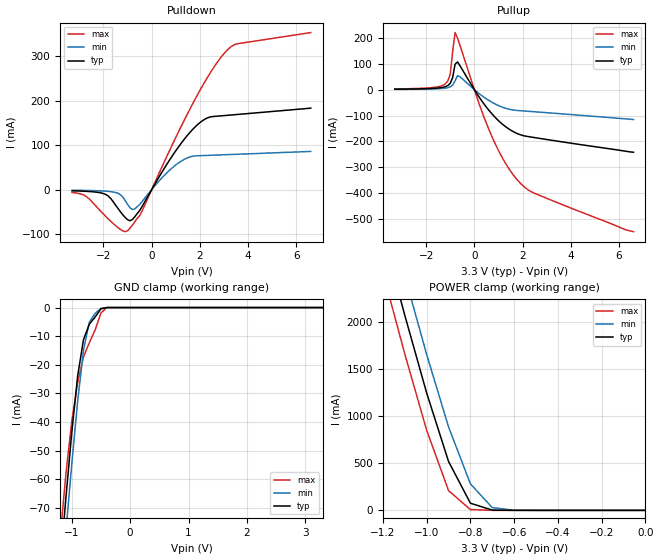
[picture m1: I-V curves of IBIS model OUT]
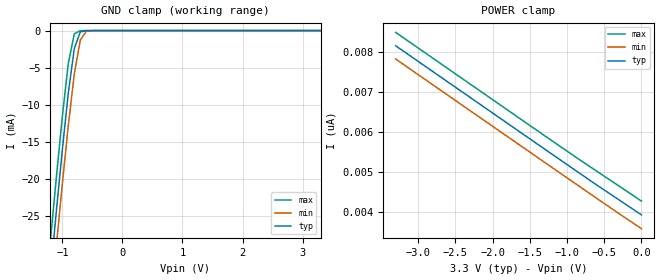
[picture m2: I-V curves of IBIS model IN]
|   TEXAS INSTRUMENTS INCORPORATED
|   Standard Linear and Logic
|   IBIS Model of SN74ALVC16334
|   16-BIT Universal Bus Driver with 3-state outputs
|   48-pin DGG, DGV, or DL Package
[IBIS Ver]   2.1
[Comment char]  |_char
[File Name]   alvc16334.ibs
[File Rev]   2.0
[Date]   9/29/98
[Source]   File originated at Texas Instruments, Inc.
[Notes]   The following is an IBIS list for the ALVC16334.
|   - This file may be incomplete or may not be fully compliant
|   with the IBIS specification. It will be replaced with a
|   version that is IBIS Revision 3.2 compliant and is complete
|   and accurate.  Please email all questions and comments to
|   sllibis@ti.com.
|   - All test data contained in this file are derived from
|   hspice(tm) simulations.
|   - File created by David Yaeger, SLL Applications
[Disclaimer]
* Property of Texas Instruments Incorporated.  Unauthorized *
* reproduction and/or distribution is strictly prohibited. *
* This product is protected under copyright law. *
* Created 1997, (C) Copyright 1997, Texas Instruments Inc., *
* All Rights Reserved *
* UNLESS THERE IS A SIGNED, WRITTEN AGREEMENT TO THE *
* CONTRARY, TEXAS INSTRUMENTS ("TI") IS PROVIDING THE IBIS *
* MODELS "AS IS" AND WITHOUT ANY WARRANTY, EXPRESSED OR *
* IMPLIED.  TI assumes no liability for: *
* 1) the accuracy of the IBIS models provided to your *
* company; *
* 2) the proper functioning of these IBIS models in your *
* design or for any resulting applications; or *
* 3) infringement of patents, copyrights or intellectual *
* property rights resulting from your use of these *
* IBIS models. *
* TI provides IBIS Models as a service to our customers. *
* You and your company shall not distribute, sell or give *
* these models to anyone else without prior written *
* permission from TI. *
* TI reserves the right to make changes to our products or *
* to discontinue any semiconductor product or service *
* without notice, and advises our customers to obtain the *
* latest version of relevant information to verify, before *
* placing orders, that the information being relied on is *
* current. *
* Please be aware that your receipt and use of the IBIS *
* information provided shall serve as acceptance of these *
* terms and conditions.  If you do not accept these terms, *
* you should return or destroy the IBIS models and any *
* other accompanying information immediately. *
[Component]   ALVC16334_DGG
[Manufacturer]  Texas Instruments, Inc.
[Package]
|   typ   min   max
R_pkg   0.056   0.039   0.068
L_pkg   3.39nH   3.078nH   3.995nH
C_pkg   0.52pF   0.414pF   0.668pF
[Pin]   signal_name   model_name   R_pin   L_pin   C_pin
1   OE_BAR   NC   0.039   3.987nH   0.654pF
2   Y1   OUT   0.047   3.725nH   0.659pF
3   Y2   OUT   0.059   3.692nH   0.604pF
4   GND   GND   0.068   3.675nH   0.606pF
5   Y3   OUT   0.055   3.473nH   0.547pF
6   Y4   OUT   0.056   3.402nH   0.497pF
7   VCC   POWER   0.057   3.3nH   0.492pF
8   Y5   OUT   0.056   3.189nH   0.455pF
9   Y6   OUT   0.058   3.154nH   0.449pF
10   GND   GND   0.058   3.094nH   0.436pF
11   Y7   OUT   0.058   3.078nH   0.424pF
12   Y8   OUT   0.06   3.081nH   0.414pF
13   Y9   OUT   0.061   3.097nH   0.416pF
14   Y10   OUT   0.06   3.126nH   0.427pF
15   GND   GND   0.061   3.158nH   0.44pF
16   Y11   OUT   0.058   3.173nH   0.45pF
17   Y12   OUT   0.056   3.189nH   0.455pF
18   VCC   POWER   0.056   3.265nH   0.49pF
19   Y13   OUT   0.054   3.322nH   0.492pF
20   Y14   OUT   0.052   3.388nH   0.544pF
21   GND   GND   0.064   3.591nH   0.605pF
22   Y15   OUT   0.059   3.677nH   0.612pF
23   Y16   OUT   0.046   3.678nH   0.668pF
24   NC   NC   0.041   3.979nH   0.659pF
25   LE_BAR   NC   0.04   3.995nH   0.658pF
26   A16   IN   0.046   3.69nH   0.662pF
27   A15   IN   0.057   3.649nH   0.602pF
28   GND   GND   0.066   3.615nH   0.602pF
29   A14   IN   0.055   3.447nH   0.547pF
30   A13   IN   0.054   3.326nH   0.492pF
31   VCC   POWER   0.055   3.239nH   0.488pF
32   A12   IN   0.056   3.183nH   0.454pF
33   A11   IN   0.057   3.144nH   0.447pF
34   GND   GND   0.058   3.099nH   0.436pF
35   A10   IN   0.059   3.086nH   0.425pF
36   A9   IN   0.06   3.081nH   0.414pF
37   A8   IN   0.061   3.097nH   0.415pF
38   A7   IN   0.06   3.119nH   0.427pF
39   GND   GND   0.06   3.144nH   0.439pF
40   A6   IN   0.056   3.13nH   0.446pF
41   A5   IN   0.057   3.208nH   0.456pF
42   VCC   POWER   0.056   3.247nH   0.487pF
43   A4   IN   0.054   3.328nH   0.491pF
44   A3   IN   0.053   3.413nH   0.546pF
45   GND   GND   0.066   3.609nH   0.606pF
46   A2   IN   0.058   3.689nH   0.607pF
47   A1   IN   0.047   3.727nH   0.662pF
48   CLK   NC   0.04   3.978nH   0.655pF
[Component]   ALVC16334_DGV
[Manufacturer]  Texas Instruments, Inc.
[Package]
|   typ   min   max
R_pkg   0.063   0.043   0.09
L_pkg   3.077nH   2.377nH   4.305nH
C_pkg   0.387pF   0.281pF   0.565pF
[Pin]   signal_name   model_name   R_pin   L_pin   C_pin
1   OE_BAR   NC   0.082   4.277nH   0.562pF
2   Y1   OUT   0.09   4.02nH   0.554pF
3   Y2   OUT   0.087   3.719nH   0.478pF
4   GND   GND   0.087   3.456nH   0.417pF
5   Y3   OUT   0.076   3.207nH   0.411pF
6   Y4   OUT   0.044   2.929nH   0.39pF
7   VCC   POWER   0.046   2.803nH   0.335pF
8   Y5   OUT   0.047   2.683nH   0.321pF
9   Y6   OUT   0.048   2.579nH   0.311pF
10   GND   GND   0.049   2.505nH   0.302pF
11   Y7   OUT   0.048   2.4nH   0.289pF
12   Y8   OUT   0.051   2.4nH   0.283pF
13   Y9   OUT   0.051   2.4nH   0.283pF
14   Y10   OUT   0.05   2.433nH   0.291pF
15   GND   GND   0.048   2.46nH   0.298pF
16   Y11   OUT   0.048   2.585nH   0.312pF
17   Y12   OUT   0.046   2.652nH   0.319pF
18   VCC   POWER   0.045   2.787nH   0.336pF
19   Y13   OUT   0.046   2.962nH   0.394pF
20   Y14   OUT   0.074   3.208nH   0.409pF
21   GND   GND   0.087   3.488nH   0.417pF
22   Y15   OUT   0.087   3.741nH   0.478pF
23   Y16   OUT   0.089   3.99nH   0.546pF
24   NC   NC   0.084   4.305nH   0.557pF
25   LE_BAR   NC   0.082   4.286nH   0.565pF
26   A16   IN   0.086   3.933nH   0.554pF
27   A15   IN   0.086   3.699nH   0.475pF
28   GND   GND   0.089   3.522nH   0.42pF
29   A14   IN   0.079   3.234nH   0.413pF
30   A13   IN   0.043   2.88nH   0.385pF
31   VCC   POWER   0.045   2.779nH   0.332pF
32   A12   IN   0.045   2.636nH   0.317pF
33   A11   IN   0.047   2.553nH   0.309pF
34   GND   GND   0.048   2.468nH   0.298pF
35   A10   IN   0.05   2.424nH   0.29pF
36   A9   IN   0.05   2.377nH   0.281pF
37   A8   IN   0.05   2.387nH   0.281pF
38   A7   IN   0.05   2.431nH   0.29pF
39   GND   GND   0.048   2.475nH   0.299pF
40   A6   IN   0.048   2.557nH   0.309pF
41   A5   IN   0.047   2.671nH   0.319pF
42   VCC   POWER   0.046   2.804nH   0.334pF
43   A4   IN   0.044   2.935nH   0.39pF
44   A3   IN   0.074   3.203nH   0.412pF
45   GND   GND   0.085   3.444nH   0.416pF
46   A2   IN   0.085   3.723nH   0.477pF
47   A1   IN   0.09   4.012nH   0.547pF
48   CLK   NC   0.083   4.288nH   0.558pF
[Component]   ALVC16334_DL
[Manufacturer]  Texas Instruments, Inc.
[Package]
|   typ   min   max
R_pkg   0.048   0.038   0.053
L_pkg   6.046nH   5.084nH   7.968nH
C_pkg   0.813pF   0.569pF   1.157pF
[Pin]   signal_name   model_name   R_pin   L_pin   C_pin
1   OE_BAR   NC   0.046   7.968nH   1.017pF
2   Y1   OUT   0.044   7.299nH   1.157pF
3   Y2   OUT   0.043   6.765nH   1.058pF
4   GND   GND   0.041   6.269nH   0.933pF
5   Y3   OUT   0.038   5.856nH   0.829pF
6   Y4   OUT   0.046   5.802nH   0.79pF
7   VCC   POWER   0.05   5.656nH   0.738pF
8   Y5   OUT   0.053   5.5nH   0.643pF
9   Y6   OUT   0.052   5.304nH   0.606pF
10   GND   GND   0.053   5.189nH   0.583pF
11   Y7   OUT   0.051   5.084nH   0.569pF
12   Y8   OUT   0.053   5.862nH   0.833pF
13   Y9   OUT   0.053   5.862nH   0.833pF
14   Y10   OUT   0.051   5.084nH   0.569pF
15   GND   GND   0.053   5.189nH   0.583pF
16   Y11   OUT   0.052   5.304nH   0.606pF
17   Y12   OUT   0.053   5.5nH   0.643pF
18   VCC   POWER   0.05   5.656nH   0.738pF
19   Y13   OUT   0.046   5.802nH   0.79pF
20   Y14   OUT   0.038   5.856nH   0.829pF
21   GND   GND   0.041   6.269nH   0.933pF
22   Y15   OUT   0.043   6.765nH   1.058pF
23   Y16   OUT   0.044   7.299nH   1.157pF
24   NC   NC   0.046   7.968nH   1.017pF
25   LE_BAR   NC   0.046   7.968nH   1.017pF
26   A16   IN   0.044   7.299nH   1.157pF
27   A15   IN   0.043   6.765nH   1.058pF
28   GND   GND   0.041   6.269nH   0.933pF
29   A14   IN   0.038   5.856nH   0.829pF
30   A13   IN   0.046   5.802nH   0.79pF
31   VCC   POWER   0.05   5.656nH   0.738pF
32   A12   IN   0.053   5.5nH   0.643pF
33   A11   IN   0.052   5.304nH   0.606pF
34   GND   GND   0.053   5.189nH   0.583pF
35   A10   IN   0.051   5.084nH   0.569pF
36   A9   IN   0.053   5.862nH   0.833pF
37   A8   IN   0.053   5.862nH   0.833pF
38   A7   IN   0.051   5.084nH   0.569pF
39   GND   GND   0.053   5.189nH   0.583pF
40   A6   IN   0.052   5.304nH   0.606pF
41   A5   IN   0.053   5.5nH   0.643pF
42   VCC   POWER   0.05   5.656nH   0.738pF
43   A4   IN   0.046   5.802nH   0.79pF
44   A3   IN   0.038   5.856nH   0.829pF
45   GND   GND   0.041   6.269nH   0.933pF
46   A2   IN   0.043   6.765nH   1.058pF
47   A1   IN   0.044   7.299nH   1.157pF
48   CLK   NC   0.046   7.967nH   1.017pF
| Models and submodels in the file (2): OUT (3-state), IN (Input)
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|   Model ALVC16334_OUT
[Model]   OUT
Model_type   3-state
Polarity   Non-Inverting
Enable   Active-High
|Variable   typ   min   max
C_comp   7.0pF   NA   NA
[Voltage range]   3.3   3.0   3.6
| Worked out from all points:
|   slope of the pulldown table from 0 to 0.495 V, typ, clamps not added: 10.9 ohm
|   slope of the pullup table from 0 to 0.495 V, typ, clamps not added: 7.36 ohm
|   GND clamp passes 1 mA (typ) near -0.52 V on its own axis
|   POWER clamp passes 1 mA (typ) near -0.63 V on its own axis
[Pullup]   | Note: Vtable = Vcc - Voutput
|   Voltage   I(typ)   I(min)   I(max)
-3.3V     1.7mA      1mA        2.8mA
-1.2V     11.5mA     5.8mA      22.8mA
-1V       24.5mA     10.9mA     60.01mA
-900mV    46.68mA    17.53mA    148mA
-800mV    98.42mA    34.15mA    220.6mA
-700mV    107.1mA    53.45mA    199.3mA
-600mV    92.82mA    50.22mA    171.6mA
600mV     -79.52mA   -41.73mA   -153.4mA
1.2V      -136.3mA   -69.07mA   -270mA
1.8V      -170.6mA   -80.67mA   -350.9mA
2.5V      -185.4mA   -85.56mA   -400.8mA
6.6V      -242mA     -115.5mA   -548.8mA
[Pulldown]
|   Voltage   I(typ)   I(min)   I(max)
-3.3V     -2.523mA   -1.255mA   -6.217mA
-2.7V     -3.72mA    -1.71mA    -15.66mA
-1.9V     -10.77mA   -3.325mA   -60.13mA
-1.3V     -49.18mA   -11.05mA   -88.98mA
-1V       -67.21mA   -32.84mA   -92.31mA
-700mV    -60.66mA   -43.17mA   -72.11mA
800mV     71.29mA    46.5mA     94.49mA
1.7V      135.3mA    75.09mA    192.6mA
2.3V      160.9mA    76.98mA    250.7mA
3.1V      166.8mA    78.63mA    311.4mA
3.5V      168.6mA    79.46mA    327mA
6.6V      183.1mA    86mA       352.8mA
[POWER_Clamp]   | Note: Vtable = Vcc - Voutput
|   Voltage   I(typ)   I(min)   I(max)
-3.3V     22.55A     22.92A     22.19A
-1.2V     2.935A     3.354A     2.523A
-1.1V     2.069A     2.487A     1.659A
-1V       1.245A     1.653A     850.2mA
-900mV    518.9mA    885.7mA    209.9mA
-800mV    75.77mA    281.1mA    8.953mA
-700mV    2.801mA    29.05mA    160uA
-600mV    75.4uA     1.568mA    1.514uA
0V        990pA      903.2pA    1.08nA
[GND_Clamp]
|   Voltage   I(typ)   I(min)   I(max)
-3.3V     -640.3mA   -651.6mA   -629.4mA
-1.2V     -90.31mA   -102.4mA   -80.27mA
-1.1V     -66.22mA   -78.02mA   -57.91mA
-1V       -43.5mA    -54.54mA   -39.6mA
-900mV    -23.93mA   -32.78mA   -26.27mA
-800mV    -11.24mA   -14.93mA   -17.28mA
-700mV    -5.815mA   -5.06mA    -12.29mA
-600mV    -3.276mA   -2.035mA   -7.795mA
-500mV    -416.4uA   -247.1uA   -1.885mA
-400mV    -9.992nA   -367.3nA   -984.6pA
3.3V      990pA      123.6nA    930pA
[Ramp]
| variable   typ   min   max
dV/dt_r   1.7364E+00/1.9231E-10  1.3957E+00/2.9903E-10  2.0142E+00/1.7016E-10
dV/dt_f   1.6302E+00/2.0099E-10  1.3593E+00/4.4330E-10  1.8600E+00/1.6534E-10
|   Model ALVC16334_IN
[Model]   IN
Model_type   Input
Polarity   Non-Inverting
Vinl = 0.8V
Vinh = 2.0V
|Variable   typ   min   max
C_comp   6pF   NA   NA
[Voltage Range]   3.3   3.0   3.6
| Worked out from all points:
|   GND clamp passes 1 mA (typ) near -0.74 V on its own axis
[POWER_Clamp]   | Note: Vtable = Vcc - Voutput
|   Voltage   I(typ)   I(min)   I(max)
-3.3V     8.169nA    7.835nA    8.505nA
-1V       5.186nA    4.852nA    5.523nA
-600mV    4.672nA    4.336nA    5.018nA
0V        3.921nA    3.575nA    4.268nA
[GND_Clamp]
|   Voltage   I(typ)   I(min)   I(max)
-3.3V     -226.9mA   -231.1mA   -222.8mA
-1.2V     -33.05mA   -37.73mA   -28.48mA
-1.1V     -24.41mA   -29.09mA   -19.85mA
-1V       -16.09mA   -20.7mA    -11.63mA
-900mV    -8.415mA   -12.77mA   -4.423mA
-800mV    -2.415mA   -5.819mA   -431.6uA
-700mV    -180.1uA   -1.262mA   -9.285uA
-600mV    -6.422uA   -95.7uA    -168.7nA
-500mV    -216.5nA   -5.198uA   -3.949nA
3.3V      3.921nA    3.952nA    3.894nA
